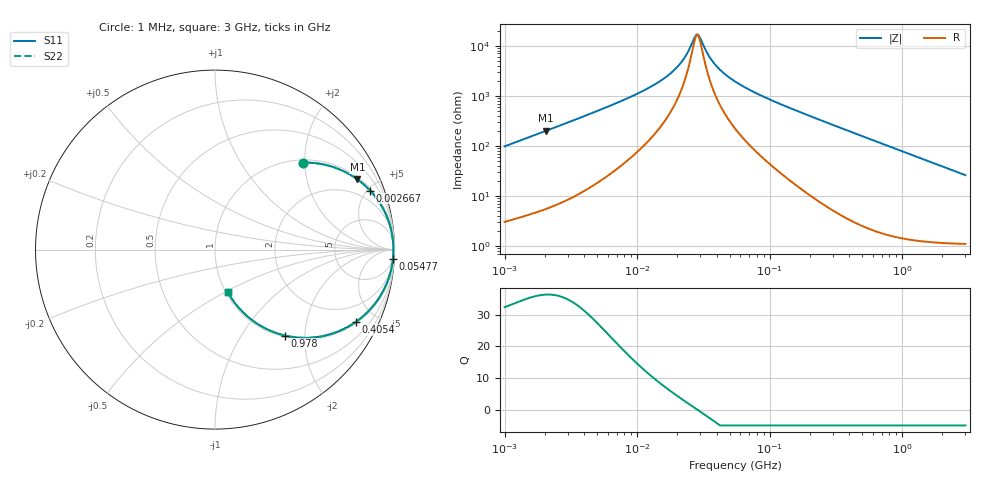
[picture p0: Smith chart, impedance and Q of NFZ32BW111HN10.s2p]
! NFZ32BW111HN10
# Hz S RI R 50
!Freq.(Hz) S11(Real) S11(Imag) S21(Real) S21(Imag) S12(Real) S12(Imag) S22(Real) S22(Imag)
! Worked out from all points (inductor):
!   401 points, 1 MHz to 3 GHz, reference 50 ohm
!   read as one part in series: L = 15.5 uH near 1.041 MHz
!   highest Q = 36.3 at 2.056 MHz (marker M1), where L = 15.5 uH
!   self-resonance near 28.29 MHz
!   S11 on the Smith chart (normalised r, x): 1 MHz: 1.06, +1.95; 2.667 MHz: 1.15, +5.19; 54.77 MHz: 5, -38; 405.4 MHz: 1.07, -3.86; 978 MHz: 1.03, -1.59; 3 GHz: 1.02, -0.52
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1000000  0.4886 0.4847  0.5114 -0.4847  0.5114 -0.4847  0.4886 0.4847
2055611  0.7932 0.3915  0.2068 -0.3915  0.2068 -0.3915  0.7932 0.3915
2666535  0.864 0.3291  0.136 -0.3291  0.136 -0.3291  0.864 0.3291
3823119  0.927 0.2449  0.073 -0.2449  0.073 -0.2449  0.927 0.2449
8686058  0.9823 0.1058  0.0177 -0.1058  0.0177 -0.1058  0.9823 0.1058
1.461624e7  0.9913 0.0515  0.00871 -0.0515  0.00871 -0.0515  0.9913 0.0515
2.095589e7  0.9936 0.0224  0.00645 -0.0224  0.00645 -0.0224  0.9936 0.0224
2.362996e7  0.9939 0.0134  0.00611 -0.0134  0.00611 -0.0134  0.9939 0.0134
2.718395e7  0.9941 0.00325  0.00593 -0.00325  0.00593 -0.00325  0.9941 0.00325
2.829425e7  0.9941 0.000363  0.00591 -0.000363  0.00591 -0.000363  0.9941 0.000363
2.944989e7  0.9941 -0.00253  0.00592 0.00253  0.00592 0.00253  0.9941 -0.00253
3.387922e7  0.9939 -0.0127  0.00607 0.0127  0.00607 0.0127  0.9939 -0.0127
3.820236e7  0.9936 -0.0216  0.00637 0.0216  0.00637 0.0216  0.9936 -0.0216
4.483659e7  0.9929 -0.034  0.00707 0.034  0.00707 0.034  0.9929 -0.034
5.477226e7  0.9915 -0.0507  0.0085 0.0507  0.0085 0.0507  0.9915 -0.0507
9.216659e7  0.9829 -0.1046  0.0171 0.1046  0.0171 0.1046  0.9829 -0.1046
2.094008e8  0.9295 -0.2438  0.0705 0.2438  0.0705 0.2438  0.9295 -0.2438
4.0536e8  0.7844 -0.4029  0.2156 0.4029  0.2156 0.4029  0.7844 -0.4029
8.005644e8  0.4869 -0.4916  0.5131 0.4916  0.5131 0.4916  0.4869 -0.4916
9.779672e8  0.3902 -0.4789  0.6098 0.4789  0.6098 0.4789  0.3902 -0.4789
1.67892e9  0.1833 -0.3743  0.8167 0.3743  0.8167 0.3743  0.1833 -0.3743
3e9  0.072 -0.2382  0.928 0.2382  0.928 0.2382  0.072 -0.2382
